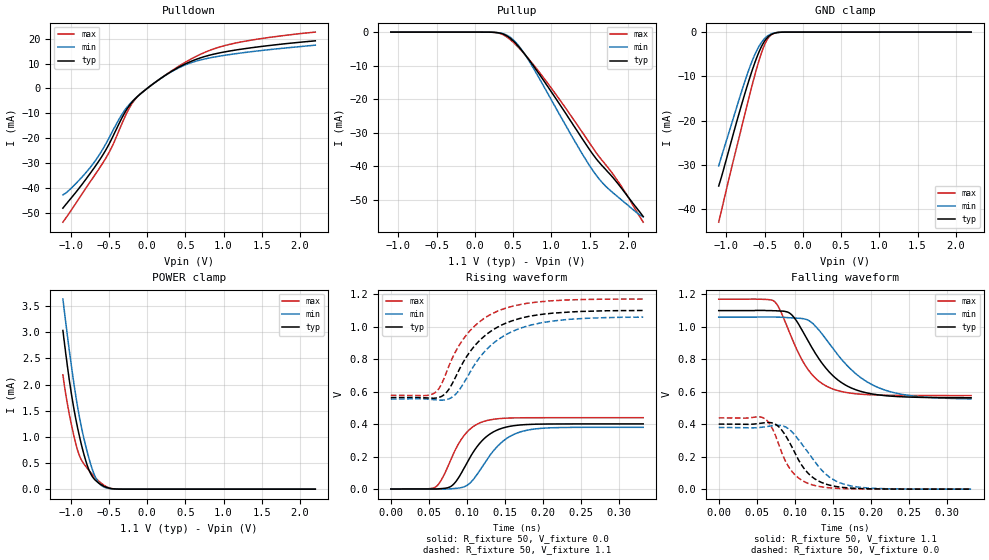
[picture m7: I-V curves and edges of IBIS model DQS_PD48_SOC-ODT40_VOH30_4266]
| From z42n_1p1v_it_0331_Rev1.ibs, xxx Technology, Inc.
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| DQS_PD48_SOC-ODT40_VOH30_4266
| (48 Ohm Pulldown, 40 Ohm System ODT Setting, VOH=VDDQ/3.0, 3200-4266Mbps)
[Model]   DQS_PD48_SOC-ODT40_VOH30_4266
Model_type   I/O
Vinl = 123.333mV
Vinh = 243.333mV
Vmeas = 183.333mV
Vref = 0.0mV
Cref = 0.0pF
Rref = 40.000Ohm
|   typ   min   max
|C_comp   0.849pF   0.799pF   0.899pF
C_comp_pullup   0.4245pF   0.3995pF   0.4495pF
C_comp_pulldown   0.4245pF   0.3995pF   0.4495pF
| Note: C_comp changes when the ODT circuit is enabled.
[Model Spec]
| Input threshold voltage corners
Vinl   0.1233V   0.1167V   0.1350V
Vinh   0.2433V   0.2367V   0.2550V
| Measurement voltage corners
Vmeas   0.1833V   0.1767V   0.1950V
| Timing spec test load voltage corners
Vref   0.0000V   0.0000V   0.0000V
| Dynamic Overshoot Parameters from LPDDR4 Specification
D_overshoot_ampl_h   0.30   NA   NA
D_overshoot_ampl_l   0.30   NA   NA
D_overshoot_area_h   0.1n   NA   NA
D_overshoot_area_l   0.1n   NA   NA
[Voltage Range]   1.1000V   1.0600V   1.1700V
[Pullup Reference]   1.1000V   1.0600V   1.1700V
| Junction Temperature (Ambient temp is 35C typ 95C min -40C max)
[Temperature Range]   50.0   110.0   -40.0
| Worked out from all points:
|   slope of the pulldown table from 0 to 0.165 V, typ, clamps not added: 43.8 ohm
|   slope of the pullup table from 0 to 0.165 V, typ, clamps not added: 13 kohm
|   GND clamp passes 1 mA (typ) near -0.45 V on its own axis
|   POWER clamp passes 1 mA (typ) near -0.88 V on its own axis
|   rising waveform, R_fixture 50, V_fixture 0.0: 20-80 % time 34.7ps typ, 38.8ps min, 30.2ps max; typ from 0.001 V to 0.401 V
|   falling waveform, R_fixture 50, V_fixture 1.1: 20-80 % time 49.3ps typ, 61.2ps min, 39.2ps max; typ from 1.1 V to 0.563 V
|   rising waveform, R_fixture 50, V_fixture 1.1: 20-80 % time 55.5ps typ, 58.1ps min, 51.7ps max; typ from 0.563 V to 1.1 V
|   falling waveform, R_fixture 50, V_fixture 0.0: 20-80 % time 32.5ps typ, 40ps min, 27.6ps max; typ from 0.401 V to 0.001 V
[Pulldown]
|   Voltage   I(typ)   I(min)   I(max)
-1.1V     -48.22mA   -42.85mA   -53.87mA
-918.5mV  -41.36mA   -37.93mA   -45.72mA
-694.1mV  -32.1mA    -29.86mA   -35.4mA
-479.6mV  -21.39mA   -18.92mA   -24.8mA
-324.5mV  -11.65mA   -10.29mA   -13.91mA
-199.1mV  -5.64mA    -5.359mA   -6.219mA
-113.3mV  -2.927mA   -2.884mA   -2.961mA
45.1mV    1.047mA    1.044mA    1.045mA
447.7mV   9.071mA    8.78mA     9.581mA
883.3mV   13.89mA    12.68mA    16.05mA
1.355V    16.35mA    14.77mA    19.42mA
2.2V      19.18mA    17.44mA    22.7mA
[GND Clamp]
|   Voltage   I(typ)   I(min)   I(max)
-1.1V     -34.74mA   -30.21mA   -42.91mA
-941.6mV  -25.02mA   -21.26mA   -31.32mA
-799.7mV  -16.31mA   -13.32mA   -21.42mA
-723.8mV  -11.94mA   -9.348mA   -16.1mA
-667.7mV  -8.907mA   -6.722mA   -12.29mA
-591.8mV  -5.255mA   -3.789mA   -7.493mA
-522.5mV  -2.665mA   -1.902mA   -3.811mA
-469.7mV  -1.357mA   -985.1uA   -1.788mA
-416.9mV  -596.7uA   -440.1uA   -664.7uA
-354.2mV  -178.1uA   -134.8uA   -159.9uA
-235.4mV  -8.186uA   -7.681uA   -4.491uA
2.2V      0A         0A         0A
[Pullup]
|   Voltage   I(typ)   I(min)   I(max)
-1.1V     6.275uA    9.671uA    2.829uA
229.9mV   -45.14uA   -46.16uA   -46.64uA
335.5mV   -340.5uA   -282.4uA   -468.8uA
431.2mV   -1.333mA   -1.089mA   -1.693mA
543.4mV   -3.63mA    -3.312mA   -3.978mA
685.3mV   -7.607mA   -7.806mA   -7.548mA
955.9mV   -16.38mA   -18.46mA   -15.4mA
1.378V    -30.95mA   -35.41mA   -29.04mA
1.589V    -37.92mA   -42.84mA   -36.13mA
1.708V    -41mA      -45.97mA   -39.55mA
1.893V    -45.92mA   -49.65mA   -45.31mA
2.2V      -55.05mA   -55.15mA   -56.74mA
[POWER Clamp]
|   Voltage   I(typ)   I(min)   I(max)
-1.1V     3.033mA    3.633mA    2.184mA
-1.044V   2.381mA    2.967mA    1.653mA
-981.2mV  1.753mA    2.275mA    1.183mA
-915.2mV  1.224mA    1.639mA    781.4uA
-855.8mV  837.6uA    1.171mA    552.2uA
-776.6mV  434.3uA    683.3uA    390.2uA
-710.6mV  232.2uA    359uA      273.1uA
-657.8mV  146.8uA    178.8uA    190.6uA
-591.8mV  77.9uA     64.81uA    105.5uA
-489.5mV  17.75uA    10.81uA    22.48uA
-380.6mV  1.603uA    1.131uA    1.341uA
2.2V      0A         0A         0A
[Ramp]
|   typ   min   max
| 20% - 80%
dV/dt_r   240.28m/34.75p   227.83m/38.76p   263.33m/30.20p
dV/dt_f   322.12m/49.32p   302.17m/61.19p   355.99m/39.15p
| 25% - 75%
|dV/dt_r   200.24m/27.67p   189.86m/30.88p   219.44m/23.94p
|dV/dt_f   268.43m/39.31p   251.80m/48.83p   296.66m/31.17p
R_load = 50
[Rising Waveform]
R_fixture = 50
V_fixture = 0.0
|   Time   V(typ)   V(min)   V(max)
0s        619.1uV    536.6uV    450.1uV
60ps      1.042mV    -84.49uV   16.73mV
69ps      4.083mV    -175.8uV   78.14mV
80ps      19.77mV    2.236mV    193.1mV
95ps      117.6mV    11.96mV    321.6mV
107ps     217.2mV    51mV       379.9mV
124ps     315.7mV    164.6mV    418.9mV
150ps     379.5mV    303.8mV    436.1mV
177ps     396.8mV    360.1mV    439mV
332ps     401.1mV    380.3mV    439.3mV
[Falling Waveform]
R_fixture   = 50
V_fixture   = 1.1
V_fixture_min = 1.06
V_fixture_max = 1.17
|   Time   V(typ)   V(min)   V(max)
0s        1.1V       1.06V      1.17V
73ps      1.099V     1.061V     1.157V
81ps      1.097V     1.059V     1.101V
94ps      1.082V     1.056V     954.9mV
115ps     934.4mV    1.046V     754.1mV
131ps     808.8mV    985mV      668.1mV
149ps     704.4mV    873.8mV    619.1mV
181ps     611.3mV    708.5mV    587.5mV
216ps     577.7mV    614.8mV    579.2mV
332ps     563.1mV    556.4mV    576.7mV
[Rising Waveform]
R_fixture   = 50
V_fixture   = 1.1
V_fixture_min = 1.06
V_fixture_max = 1.17
|   Time   V(typ)   V(min)   V(max)
0s        562.8mV    553.9mV    576.6mV
57ps      559mV      549.8mV    590mV
66ps      568.8mV    547mV      640mV
79ps      633.7mV    560.8mV    785.9mV
91ps      744.4mV    616.5mV    892.7mV
109ps     874.4mV    756.8mV    997.7mV
126ps     952.2mV    859mV      1.06V
146ps     1.01V      934.9mV    1.105V
210ps     1.081V     1.032V     1.158V
332ps     1.099V     1.058V     1.169V
[Falling Waveform]
R_fixture = 50
V_fixture = 0.0
|   Time   V(typ)   V(min)   V(max)
0s        401.2mV    380.4mV    439.4mV
61ps      410.3mV    384.3mV    433.3mV
70ps      408.7mV    391.1mV    378.8mV
78ps      388.8mV    394mV      288.8mV
94ps      280.8mV    363.6mV    123.8mV
110ps     142.2mV    274.1mV    53.17mV
124ps     71.85mV    184.8mV    25.79mV
146ps     24.83mV    73.47mV    8.582mV
173ps     7.298mV    21.37mV    2.537mV
332ps     679.4uV    647.7uV    471uV
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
